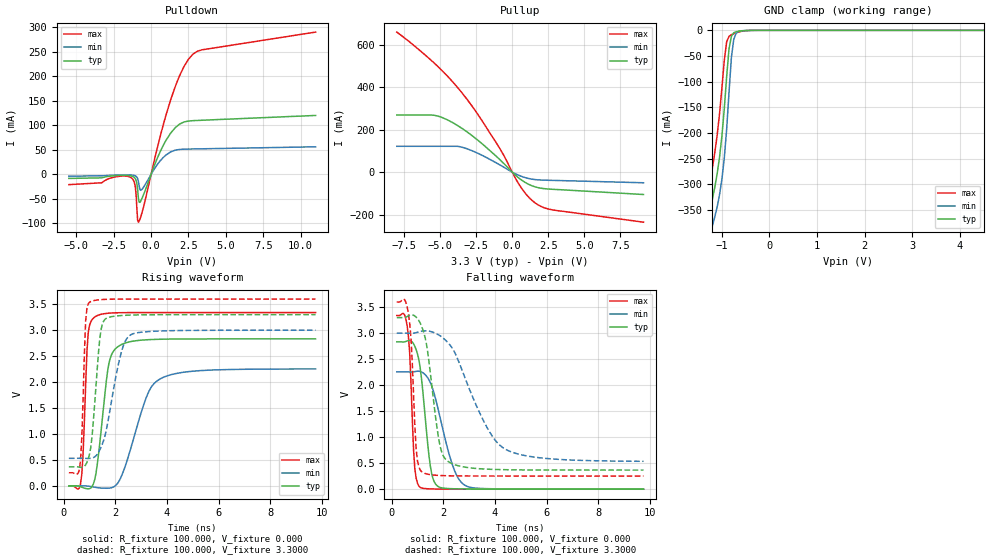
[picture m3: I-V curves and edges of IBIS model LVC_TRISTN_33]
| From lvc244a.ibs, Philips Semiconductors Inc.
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|   Model LVC_TRISTN_33
[Model]   LVC_TRISTN_33
Model_type   3-state
Polarity   Non-Inverting
Enable   Active-Low
Vmeas =  1.5000V
Cref  = 50.0000pF
Rref  =  0.5000k
Vref  =  0.000V
C_comp   3.40pF   2.95pF   3.93pF
[Model Spec]
| Note: The input and output voltage ratings may be exceeded if the input and
|   output current ratings are observed (please refer to the data sheet)
|   Subparameter   typ   min   max
| Timing Thresholds
Vmeas   1.5   1.5   1.5
|Ambient temperature:   25.0000   85.0000   -40.0000
[Temperature Range]   40.0000   100.0000   -25.0000
[Voltage Range]   3.3000V   3.0000V   3.6000V
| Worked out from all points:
|   slope of the pulldown table from 0 to 0.495 V, typ, clamps not added: 12.8 ohm
|   slope of the pullup table from 0 to 0.495 V, typ, clamps not added: 16.7 ohm
|   GND clamp passes 1 mA (typ) near -0.57 V on its own axis
|   rising waveform, R_fixture 100.000, V_fixture 0.000: 20-80 % time 380ps typ, 852ps min, 156ps max; typ from 0 V to 2.83 V
|   rising waveform, R_fixture 100.000, V_fixture 3.3000: 20-80 % time 277ps typ, 570ps min, 130ps max; typ from 0.367 V to 3.3 V
|   falling waveform, R_fixture 100.000, V_fixture 0.000: 20-80 % time 344ps typ, 701ps min, 170ps max; typ from 2.83 V to 0 V
|   falling waveform, R_fixture 100.000, V_fixture 3.3000: 20-80 % time 457ps typ, 1.33ns min, 187ps max; typ from 3.3 V to 0.367 V
|Process Range   nominal   slow   fast
[Pulldown]
| voltage   I(typ)   I(min)   I(max)
-5.5V     -8.321mA   -3.843mA   -21.05mA
-1.4V     -2.946mA   -1.211mA   -5.795mA
-1.05V    -9.131mA   -3.158mA   -26.89mA
-900mV    -31.33mA   -8.405mA   -93.71mA
-850mV    -48.34mA   -14.32mA   -97.69mA
-800mV    -56.89mA   -23.68mA   -95.44mA
-650mV    -51.7mA    -31.9mA    -82.65mA
500mV     38.92mA    23.46mA    64.5mA
1.3V      83.8mA     45.64mA    151.3mA
2.2V      106.9mA    51.35mA    220.1mA
2.8V      109.6mA    51.79mA    245.4mA
11V       120.2mA    56.22mA    290.4mA
[Pullup]
| voltage   I(typ)   I(min)   I(max)
-8V       269.1mA    121.8mA    660.4mA
-5.4V     268mA      121.8mA    514mA
-4.4V     243.3mA    121.8mA    446.3mA
-3.6V     211.5mA    119.5mA    383.9mA
-2.4V     151.5mA    89.4mA     274mA
-800mV    55.11mA    31.81mA    104.4mA
600mV     -35.22mA   -19.02mA   -71.23mA
1V        -52.59mA   -27.82mA   -107.4mA
1.6V      -69.81mA   -35.37mA   -146mA
2.2V      -77.8mA    -37.89mA   -167.8mA
2.8V      -81.05mA   -39.02mA   -178.1mA
9.1V      -105.6mA   -50.26mA   -236.2mA
[GND_clamp]
| voltage   I(typ)   I(min)   I(max)
-5.5V     -4.552A    -4.581A    -4.529A
-1.35V    -436.9mA   -483.2mA   -382.8mA
-1.3V     -392.7mA   -439.6mA   -337.9mA
-1.2V     -328.9mA   -381mA     -268.2mA
-1.05V    -247.4mA   -320.5mA   -163.3mA
-950mV    -153.3mA   -249mA     -58.72mA
-900mV    -90.37mA   -192.9mA   -22.55mA
-850mV    -36.04mA   -120.8mA   -11.79mA
-800mV    -11.48mA   -52.5mA    -8.579mA
-750mV    -4.615mA   -17.21mA   -6.53mA
-700mV    -2.665mA   -5.464mA   -4.804mA
5.5V      991.5pA    8.054nA    37.33pA
[Ramp]
| variable   typ   min   max
dV/dt_r   1.700V/380.528ps   1.352V/852.831ps   2.004V/156.190ps
dV/dt_f   1.760V/456.903ps   1.479V/1.332ns   2.008V/187.209ps
R_load = 100.000
[Rising Waveform]
R_fixture   = 100.000
V_fixture   = 0.000
V_fixture_min = 0.000
V_fixture_max = 0.000
| time   V(typ)   V(min)   V(max)
200ps     -36.86uV   -16.51uV   -23.98uV
650ps     -15.82mV   569.7uV    34.32mV
750ps     -34.28mV   1.178mV    615mV
950ps     -56.97mV   -5.026mV   2.951V
1.2ns     119.1mV    -25.01mV   3.254V
1.75ns    2.358V     -43.95mV   3.328V
2.15ns    2.7V       99.64mV    3.337V
3.2ns     2.815V     1.708V     3.34V
3.7ns     2.825V     2.051V     3.34V
9.75ns    2.833V     2.253V     3.34V
[Rising Waveform]
R_fixture   = 100.000
V_fixture   = 3.3000
V_fixture_min = 3.0000
V_fixture_max = 3.6000
| time   V(typ)   V(min)   V(max)
200ps     366.8mV    531.4mV    252.7mV
650ps     356.9mV    532mV      481.2mV
700ps     357mV      532.2mV    916.6mV
850ps     406.5mV    530.6mV    3.184V
1ns       609.7mV    529.3mV    3.538V
1.4ns     2.848V     697.3mV    3.588V
1.65ns    3.229V     1.079V     3.595V
2.25ns    3.283V     2.611V     3.599V
2.65ns    3.292V     2.925V     3.6V
9.75ns    3.3V       3V         3.6V
[Falling Waveform]
R_fixture   = 100.000
V_fixture   = 0.000
V_fixture_min = 0.000
V_fixture_max = 0.000
| time   V(typ)   V(min)   V(max)
200ps     2.833V     2.255V     3.34V
600ps     2.85V      2.255V     3.148V
700ps     2.859V     2.254V     2.612V
900ps     2.746V     2.261V     383.6mV
1.1ns     2.356V     2.264V     35.94mV
1.5ns     440.2mV    2.05V      5.412mV
1.8ns     51.46mV    1.539V     2.447mV
2.4ns     7.89mV     405mV      603.4uV
2.95ns    3.509mV    49.42mV    167.7uV
9.75ns    -706nV     101.4uV    2.872pV
[Falling Waveform]
R_fixture   = 100.000
V_fixture   = 3.3000
V_fixture_min = 3.0000
V_fixture_max = 3.6000
| time   V(typ)   V(min)   V(max)
200ps     3.3V       3V         3.6V
650ps     3.333V     2.999V     3.378V
750ps     3.353V     2.998V     2.908V
950ps     3.309V     3.01V      773.9mV
1.2ns     3.081V     3.04V      321.6mV
1.85ns    895.6mV    2.958V     263.6mV
2.2ns     528.2mV    2.807V     257.5mV
3.7ns     384.8mV    1.18V      252.9mV
4.4ns     374.4mV    769.8mV    252.8mV
9.75ns    366.9mV    536.4mV    252.7mV
